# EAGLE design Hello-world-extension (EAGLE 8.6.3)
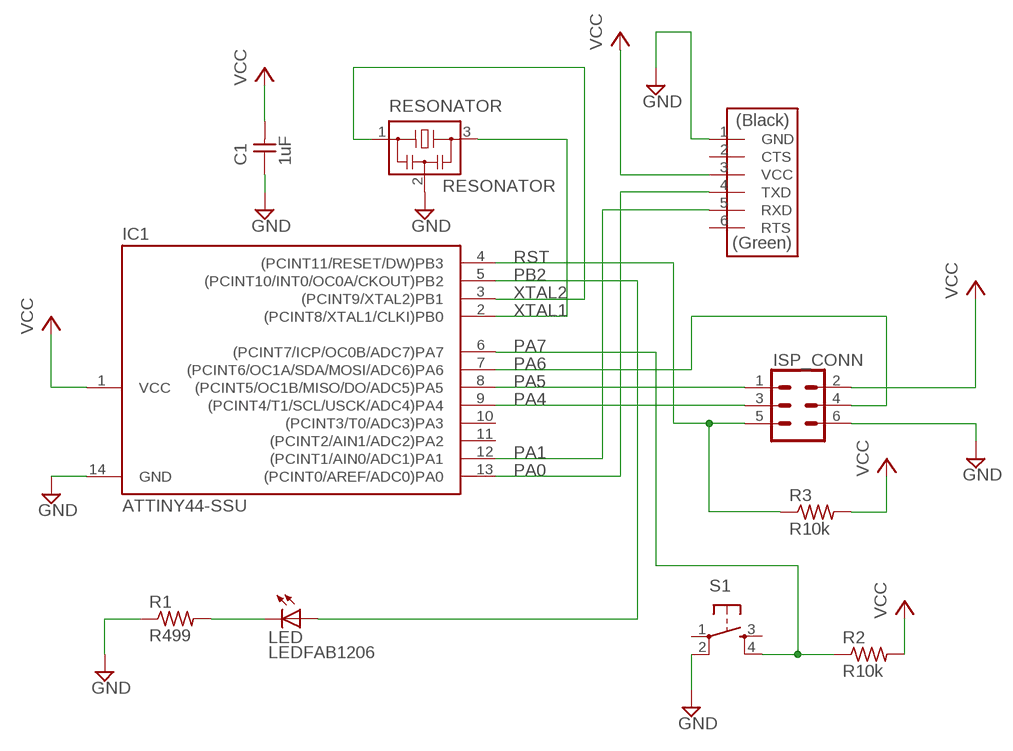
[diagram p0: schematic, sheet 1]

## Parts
C1  1uF  CAP-UNPOLARIZED  [C1206]
IC1  ATTINY44-SSU  [SOIC14]
ISP_CONN  CONN_03X2FEMALE_SMD  [2X3_SMD]
LED  LEDFAB1206  [LED1206FAB]
R1  R499  RES-US1206FAB  [R1206FAB]
R2  R10k  RES-US1206FAB  [R1206FAB]
R3  R10k  RES-US1206FAB  [R1206FAB]
RESONATOR  RESONATOR  [EFOBM]
S1  6MM_SWITCH6MM_SWITCH  [6MM_SWITCH]
U$3  FTDI-SMD-HEADER  [1X06SMD]

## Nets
GND: C1.1 IC1.14(GND) ISP_CONN.6 R1.1 RESONATOR.2 S1.2(P1) U$3.1(GND)
N$11: LED.2(C) R1.2
PA0: IC1.13((PCINT0/AREF/ADC0)PA0) U$3.4(TXD)
PA1: IC1.12((PCINT1/AIN0/ADC1)PA1) U$3.5(RXD)
PA4: IC1.9((PCINT4/T1/SCL/USCK/ADC4)PA4) ISP_CONN.3
PA5: IC1.8((PCINT5/OC1B/MISO/DO/ADC5)PA5) ISP_CONN.1
PA6: IC1.7((PCINT6/OC1A/SDA/MOSI/ADC6)PA6) ISP_CONN.4
PA7: IC1.6((PCINT7/ICP/OC0B/ADC7)PA7) R2.1 S1.4(S1)
PB2: IC1.5((PCINT10/INT0/OC0A/CKOUT)PB2) LED.1(A)
RST: IC1.4((PCINT11/RESET/DW)PB3) ISP_CONN.5 R3.1
VCC: C1.2 IC1.1(VCC) ISP_CONN.2 R2.2 R3.2 U$3.3(VCC)
XTAL1: IC1.2((PCINT8/XTAL1/CLKI)PB0) RESONATOR.3
XTAL2: IC1.3((PCINT9/XTAL2)PB1) RESONATOR.1
Unconnected: IC1.10((PCINT3/T0/ADC3)PA3) IC1.11((PCINT2/AIN1/ADC2)PA2) S1.1(P) S1.3(S) U$3.2(CTS) U$3.6(RTS)

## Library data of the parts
C1 = fab:CAP-UNPOLARIZED
IC1 = fab:ATTINY44
ISP_CONN = fab:CONN_03X2: Multi connection point. Often used as Generic Header-pin footprint for 0.1 inch spaced/style header connections You can populate with any combo of single row headers, but if you'd like an exact match, check these: Header - 2x3 (Male, 0.1") (PRT-12807) Header - 2x3 (Female, 0.1") (PRT-13010) 2x3 Pin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; PROD_ID: CONN-11290
LED = fab:LED: LED
R1-R3 = fab:RES-US: Resistor (US Symbol)
RESONATOR = fab:RESONATOR
S1 = fab:6MM_SWITCH: OMRON SWITCH
U$3 = fab:FTDI-SMD-HEADER

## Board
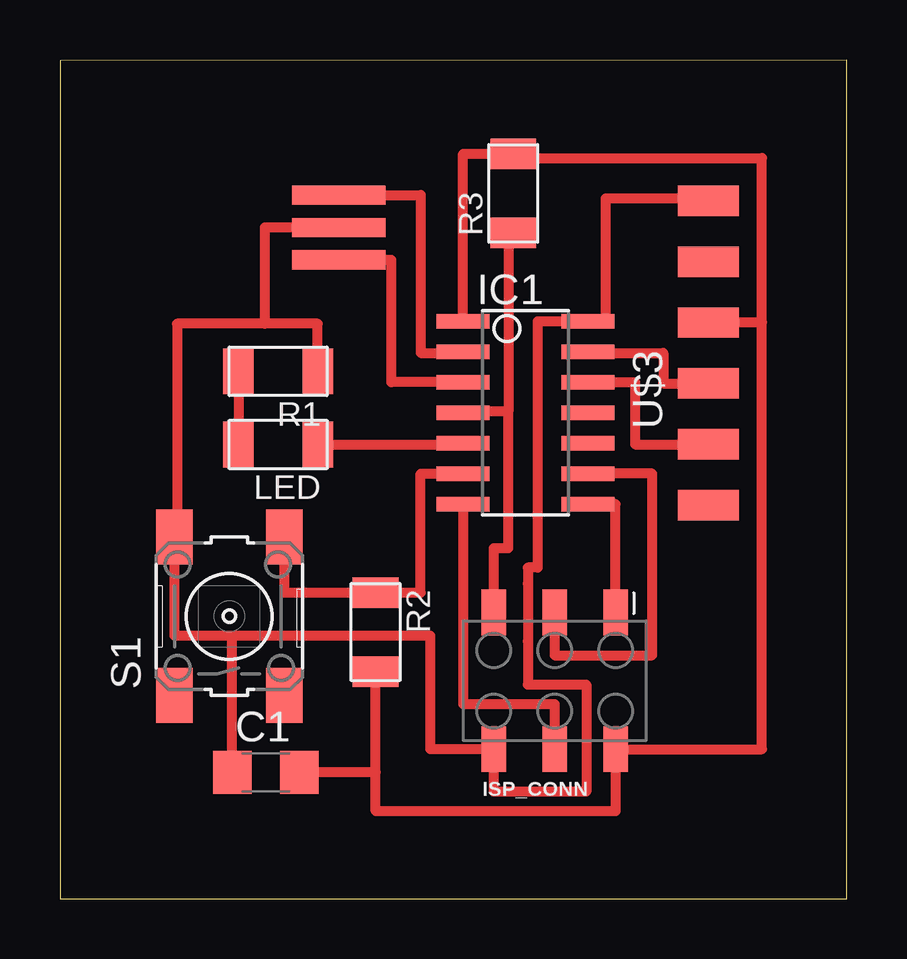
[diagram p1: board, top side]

Size 32.8 x 34.98 mm. Coordinates in mm from the lower left corner, seen from the top.
Outline: 0,0 32.8,0 32.8,34.98 0,34.95 0,0
Copper layers (1*16): Top 0.035mm / dielectric 1.5mm / Bottom 0.035mm
Design rules "default *": minimum track width 16mil, minimum drill 0.35mm, track to track 16mil, track to pad 16mil, pad to pad 16mil, via to via 16mil, smd to smd 16mil, copper to edge 40mil, drill to drill 6mil, minimum pad ring 10mil, minimum via ring 8mil, stop-mask expansion 4mil, vias tented up to drill 0mil, thermal gap 10mil

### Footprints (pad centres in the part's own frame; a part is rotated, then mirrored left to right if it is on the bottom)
C1206 = smd 1.6 x 1.8: 1 -1.4,0; 2 1.4,0
SOIC14 = smd 0.61 x 2.21: 1 -3.81,-2.603; 2 -2.54,-2.603; 3 -1.27,-2.603; 4 0,-2.603; 5 1.27,-2.603; 6 2.54,-2.603; 7 3.81,-2.603; 8 3.81,2.603; 9 2.54,2.603; 10 1.27,2.603; 11 0,2.603; 12 -1.27,2.603; 13 -2.54,2.603; 14 -3.81,2.603
2X3_SMD = smd 1.02 x 1.9: 1 -2.54,-2.85; 2 -2.54,2.85; 3 0,-2.85; 4 0,2.85; 5 2.54,-2.85; 6 2.54,2.85
LED1206FAB = smd 1.27 x 1.905: 1 -1.651,0; 2 1.651,0
R1206FAB = smd 1.27 x 1.905: 1 -1.651,0; 2 1.651,0
EFOBM = smd 0.8 x 3.9: 1 -1.35,0; 2 0,0; 3 1.35,0
6MM_SWITCH = smd 2.286 x 1.524: 1 -3.302,2.286; 2 3.302,2.286; 3 -3.302,-2.286; 4 3.302,-2.286
1X06SMD = smd 2.54 x 1.27: 1 0,6.35; 2 0,3.81; 3 0,1.27; 4 0,-1.27; 5 0,-3.81; 6 0,-6.35

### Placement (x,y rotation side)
C1  8.59,5.28 0 top
IC1  19.41,20.27 270 top
ISP_CONN  20.62,9.09 180 top
LED  9.09,18.95 180 top
R1  9.09,22 180 top
R2  13.16,11.13 270 top
R3  18.9,29.41 90 top
RESONATOR  11.63,27.99 90 top
S1  7.06,11.79 90 top
U$3  27.03,22.76 0 top

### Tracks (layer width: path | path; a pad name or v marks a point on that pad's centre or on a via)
GND
  Top 0.406: R1.1 10.74,23.98 8.53,23.98 | 8.53,23.98 4.88,23.98 4.88,15.09 S1.2 4.78,10.97 7.19,10.97 | U$3.1 27.03,29.21 22.76,29.21 22.76,24.08 IC1.14 19.91,24.08 19.91,13.82 19.51,13.82 19.51,13.15 19.51,10.74 19.51,8.94 21.95,8.94 21.95,4.47 18.08,4.47 ISP_CONN.6 15.44,6.24 15.44,10.97 7.19,10.97 | C1.1 7.19,10.97 | RESONATOR.2 8.53,27.99 8.53,23.98
N$11
  Top 0.406: R1.2 LED.2
PA0
  Top 0.406: IC1.13 22.06,22.76 25.15,22.76 25.15,21.49 U$3.4
PA1
  Top 0.406: IC1.12 23.98,21.54 23.98,18.95 U$3.5
PA4
  Top 0.406: ISP_CONN.3 20.62,10.16 24.69,10.16 24.69,17.73 IC1.9
PA5
  Top 0.406: ISP_CONN.1 23.16,16.46 IC1.8
PA6
  Top 0.406: IC1.7 16.8,8.13 20.62,8.13 ISP_CONN.4
PA7
  Top 0.406: S1.4 9.35,12.78 R2.1 15.04,12.78 15.04,17.73 IC1.6
PB2
  Top 0.406: LED.1 16.8,18.95 IC1.5
RST
  Top 0.406: IC1.4 16.8,20.32 18.69,20.32 | ISP_CONN.5 18.08,14.63 18.69,14.63 18.69,20.32 | R3.1 18.69,27.76 18.69,20.32
VCC
  Top 0.406: 29.26,24.03 U$3.3 | 29.26,24.03 29.26,6.24 ISP_CONN.2 23.16,3.66 13.16,3.66 13.16,5.28 | 29.26,24.03 29.26,30.89 18.9,30.89 R3.2 16.8,31.06 IC1.1 | 13.16,5.28 R2.2 | 13.16,5.28 C1.2
XTAL1
  Top 0.406: RESONATOR.3 15.04,29.34 15.04,22.76 16.8,22.76 IC1.2
XTAL2
  Top 0.406: IC1.3 13.82,21.54 13.82,26.64 RESONATOR.1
